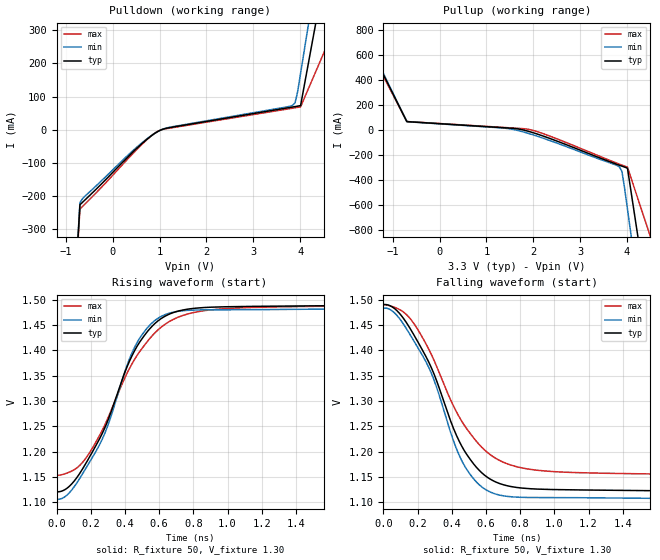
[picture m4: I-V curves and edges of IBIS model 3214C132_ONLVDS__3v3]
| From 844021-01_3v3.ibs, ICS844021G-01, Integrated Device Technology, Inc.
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[Model] 3214C132_ONLVDS__3v3
Model_type   Output
Polarity   Non-Inverting
|   typ   min   max
C_comp   2pF   1.5pF   2.5pF
Vmeas = 1.30V
Rref = 50
Cref = 0
Vref = 1.30V
|   typ   min   max
[Voltage range]   3.3V   3.135V   3.465V
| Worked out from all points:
|   slope of the pulldown table from 0 to 0.495 V, typ, clamps not added: 7.04 ohm
|   slope of the pullup table from 0 to 0.495 V, typ, clamps not added: 42.2 ohm
|   rising waveform, R_fixture 50, V_fixture 1.30: 20-80 % time 285ps typ, 262ps min, 310ps max; typ from 1.12 V to 1.49 V
|   falling waveform, R_fixture 50, V_fixture 1.30: 20-80 % time 285ps typ, 262ps min, 310ps max; typ from 1.49 V to 1.12 V
[Pulldown]
|Voltage   I (typ)   I (min)   I (max)
-3.3V     -8.39A     -7.266A    -10.27A
-1.22V    -1.479A    -1.5A      -1.457A
-591mV    -211.7mA   -200.4mA   -224mA
489.3mV   -59.32mA   -55.67mA   -63.3mA
975.4mV   -4.205mA   -4.28mA    -3.711mA
3.838V    68.61mA    73.51mA    65.02mA
3.892V    69.9mA     81.13mA    66.26mA
3.946V    71.22mA    114.1mA    67.5mA
4.01V     72.87mA    170.3mA    68.97mA
4.528V    470.8mA    626.9mA    239.4mA
5.046V    1.017A     1.085A     932.5mA
6.6V      2.661A     2.463A     3.018A
[Pullup]
|Voltage   I (typ)   I (min)   I (max)
-3.3V     2.653A     2.309A     3.233A
-1.74V    1.003A     926.2mA    1.139A
-1.22V    454.9mA    466.6mA    442.4mA
-700mV    65.2mA     65.75mA    65.81mA
1.407V    15.09mA    11.78mA    17.43mA
1.894V    -12.38mA   -29.16mA   3.491mA
3.784V    -277.2mA   -285.9mA   -268mA
3.838V    -284.6mA   -298mA     -275.8mA
3.892V    -291.8mA   -334.2mA   -283.5mA
4.01V     -307.8mA   -635.4mA   -300.1mA
4.528V    -1.584A    -2.049A    -888.8mA
6.6V      -8.402A    -7.759A    -9.545A
[Ramp]
|   typ   min   max
dV/dt_r   0.296/0.44n   0.302/0.405n   0.269/0.484n
dV/dt_f   0.296/0.44n   0.302/0.405n   0.269/0.484n
R_load =   50.0000
[Rising Waveform]
R_fixture = 50
V_fixture = 1.30   |Vcc_typ
V_fixture_min = 1.30 |Vcc_min
V_fixture_max = 1.31 |Vcc_max
C_fixture = 0.0p
| Time   typ   min   max
0s        1.121V     1.106V     1.153V
74.82ps   1.131V     1.119V     1.159V
172.4ps   1.177V     1.167V     1.187V
286.3ps   1.25V      1.239V     1.255V
406.7ps   1.363V     1.365V     1.351V
465.2ps   1.405V     1.412V     1.387V
553.1ps   1.446V     1.452V     1.426V
647.4ps   1.47V      1.472V     1.454V
1.067ns   1.486V     1.48V      1.484V
3.25ns    1.491V     1.484V     1.49V
[Falling Waveform]
R_fixture = 50
V_fixture = 1.30   |Vcc_typ
V_fixture_min = 1.30 |Vcc_min
V_fixture_max = 1.31 |Vcc_max
C_fixture = 0.0p
| Time   typ   min   max
0s        1.49V      1.483V     1.49V
74.82ps   1.48V      1.471V     1.484V
172.4ps   1.434V     1.422V     1.456V
286.3ps   1.361V     1.35V      1.388V
406.7ps   1.248V     1.224V     1.292V
465.2ps   1.206V     1.177V     1.256V
553.1ps   1.166V     1.137V     1.217V
647.4ps   1.141V     1.117V     1.189V
1.067ns   1.125V     1.109V     1.159V
3.25ns    1.121V     1.106V     1.153V
